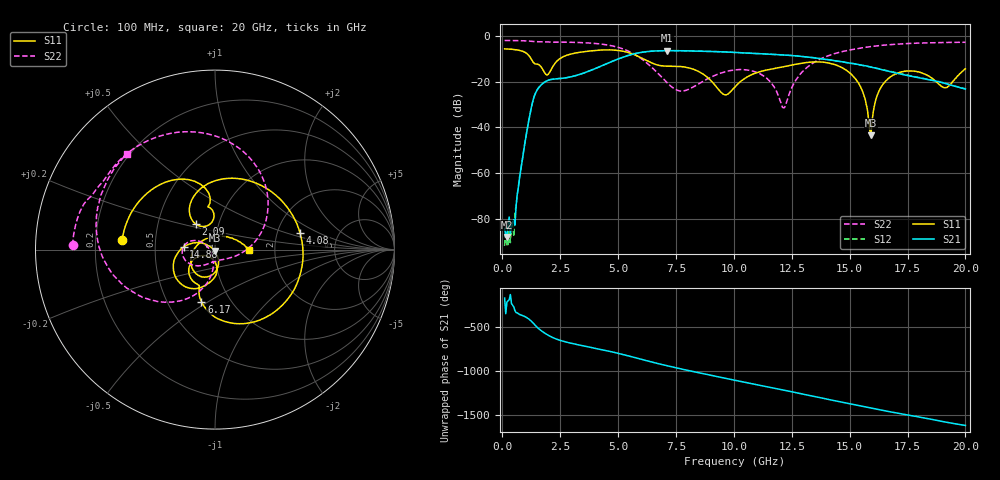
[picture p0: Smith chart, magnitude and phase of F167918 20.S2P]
!  2-Port S-parameters saved by WinCal
! VAR MeasName=S-Parameters (CALIBRATED_DATA) read from VNA (N5242A)
! VAR MeasDate=2016-11-22 10:25:44
! VAR NAME=F167918 20
! VAR FILENAME=F167918 20.S2P
! VAR DATE=2016-11-22 10:25:44
! VAR PHYS_PORTS=1,2
# Hz S DB R 50
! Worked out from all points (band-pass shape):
!   401 points, 100 MHz to 20 GHz, reference 50 ohm
!   highest |S21| = -6.46 dB at 7.115 GHz (marker M1); lowest = -87.9 dB at 199.5 MHz (marker M2)
!   |S21| within 3 dB of the highest: 5.174 GHz to 13.34 GHz (8.167 GHz wide, 88.2 % of centre)
!   lowest |S11| = -43.5 dB at 15.92 GHz (marker M3), VSWR 1.01, Z = 49.8 - j0.635 ohm
!   |S11| at or under -10 dB: 1.244 GHz to 2.483 GHz (1.239 GHz wide, 66.5 % of centre); 6.077 GHz to end of sweep
!   |S22| runs from -31.5 to -2.0 dB; largest |S21 - S12| = 0.0042
!   S11 on the Smith chart (normalised r, x): 100 MHz: 0.32, +0.05; 2.09 GHz: 0.78, +0.23; 4.08 GHz: 2.69, +0.64; 6.17 GHz: 0.73, -0.47; 14.88 GHz: 0.70, +0.02; 20 GHz: 1.47, -0.01
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1e8  -5.68 174.1  -84.13 -172.0  -91.78 174.5  -2.00 178.3
1.995e8  -5.72 168.2  -87.90 141.4  -91.98 168.6  -2.01 176.6
5.4775e8  -6.02 146.9  -82.78 44.8  -77.80 72.8  -2.06 170.7
1.34375e9  -11.66 96.1  -27.63 -98.2  -27.61 -98.4  -2.46 157.0
2.09e9  -15.08 126.9  -19.12 111.6  -19.09 111.4  -2.75 146.8
3.43325e9  -7.05 51.3  -16.54 10.5  -16.56 10.3  -2.95 121.1
4.08e9  -6.32 10.9  -14.02 -23.7  -14.03 -23.7  -3.38 104.2
5.1745e9  -6.65 -57.3  -9.46 -89.0  -9.46 -88.9  -5.57 65.3
6.1695e9  -10.47 -104.6  -6.98 -157.1  -6.96 -157.1  -11.26 20.1
6.7665e9  -12.88 -112.6  -6.52 163.1  -6.51 163.1  -16.85 -9.1
7.11475e9  -13.24 -114.8  -6.46 141.3  -6.45 141.3  -20.46 -29.1
8.30875e9  -14.80 -143.4  -6.62 71.7  -6.58 71.7  -21.99 -110.5
1.005e10  -22.26 -87.0  -7.23 -23.7  -7.24 -23.5  -14.89 -165.6
1.13435e10  -15.10 -96.7  -7.91 -92.0  -7.88 -91.7  -17.90 156.6
1.21395e10  -13.52 -106.6  -8.34 -134.4  -8.30 -134.4  -31.46 -159.3
1.338325e10  -11.46 -132.3  -9.48 157.5  -9.44 157.6  -12.12 -110.5
1.487575e10  -15.15 175.0  -11.70 77.4  -11.65 77.3  -6.42 -145.9
1.547275e10  -22.27 152.6  -12.73 45.6  -12.75 45.7  -5.32 -157.6
1.59205e10  -43.47 -108.0  -13.67 21.5  -13.65 22.1  -4.67 -166.0
1.67165e10  -18.34 -88.1  -15.50 -18.8  -15.48 -18.2  -3.86 179.9
1.915425e10  -22.63 94.5  -20.87 -137.5  -20.82 -137.2  -2.88 143.4
2e10  -14.41 -0.6  -23.25 -175.3  -23.13 -174.8  -2.80 132.7
